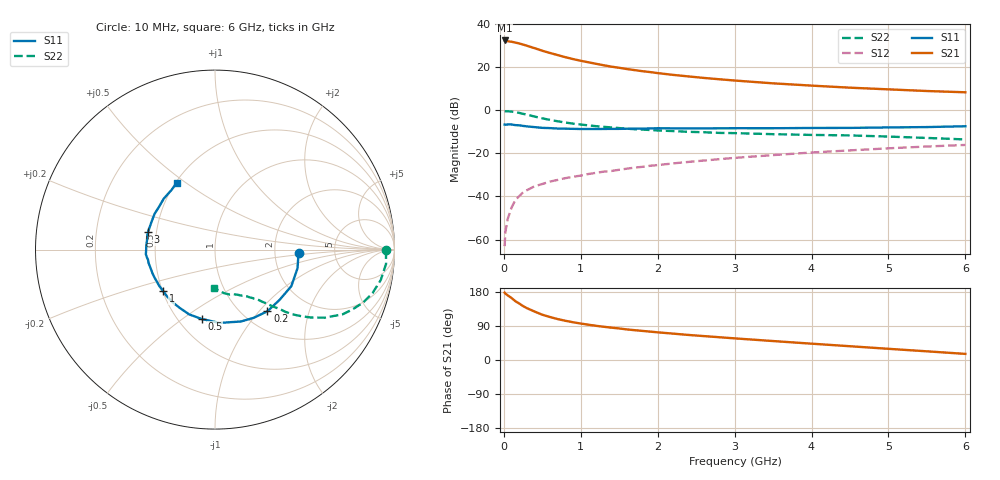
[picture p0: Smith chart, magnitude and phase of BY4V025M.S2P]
! SIEMENS Small Signal Semiconductors
! BFY420
! Si NPN RF SIEGET Grounded Emitter Transistor in MICRO-X
! VCE = 4 V  IC = 25 mA
! Common Emitter S-Parameters:  October  1996
# GHz  S  MA  R  50
!  f  S11  S21  S12  S22
! GHz  MAG  ANG  MAG  ANG  MAG  ANG  MAG  ANG
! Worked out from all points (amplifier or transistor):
!   36 points, 10 MHz to 6 GHz, reference 50 ohm
!   highest |S21| = 32.5 dB at 10 MHz (marker M1)
!   |S21| within 3 dB of that: start of sweep to 348.3 MHz
!   unconditionally stable (mu >= 1): start of sweep to 14.18 MHz; 1.92 GHz to end of sweep
!   at 250 MHz: K = 0.35, MSG = 34.3 dB, |S12| = -38.1 dB
!   at 1.4 GHz: K = 0.94, MSG = 24.2 dB, |S12| = -28.1 dB
!   at 6 GHz: K = 1.06, MAG = 10.8 dB, |S12| = -16.0 dB
!   S11 on the Smith chart (normalised r, x): 10 MHz: 2.76, -0.13; 200 MHz: 1.29, -1.11; 500 MHz: 0.65, -0.59; 1 GHz: 0.50, -0.27; 3 GHz: 0.45, +0.10; 6 GHz: 0.51, +0.46
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0.01  0.4692 -2.3  42.32 177.8  0.0007 67.7  0.9503 -0.2
0.02  0.4657 -5.1  41.78 175.2  0.0015 77.6  0.9528 -1.3
0.05  0.4714 -12.7  40.52 170.7  0.003 84.9  0.9564 -4.8
0.1  0.4716 -25.6  39.54 163.6  0.0055 79.1  0.939 -10.4
0.15  0.4558 -38.0  37.77 155.2  0.0083 74.1  0.9107 -15.4
0.2  0.4511 -49.6  36.07 149.1  0.0102 73.2  0.8772 -19.6
0.25  0.437 -60.4  33.97 142.3  0.0125 68.0  0.8348 -23.6
0.3  0.4257 -70.2  31.93 136.8  0.014 66.4  0.797 -26.9
0.4  0.4093 -86.4  27.99 127.8  0.0173 63.6  0.7197 -31.8
0.5  0.3936 -100.9  24.4 119.5  0.0195 61.5  0.6551 -35.3
0.6  0.3885 -111.8  21.66 113.4  0.0222 61.3  0.6023 -37.9
0.7  0.3795 -121.5  19.34 108.0  0.0243 61.3  0.5598 -40.0
0.8  0.3766 -129.5  17.27 103.5  0.0267 59.5  0.523 -41.5
1  0.37 -141.6  14.26 96.2  0.0306 60.3  0.4702 -43.5
1.1  0.3707 -147.1  13.15 93.1  0.0333 61.2  0.4491 -44.7
1.6  0.3752 -166.3  9.16 80.7  0.0443 60.9  0.3764 -48.8
2.2  0.3834 179.9  6.705 69.6  0.0587 59.8  0.3317 -53.7
3  0.386 165.4  4.957 57.1  0.079 55.9  0.2969 -59.8
3.5  0.3858 157.0  4.263 50.0  0.0916 52.7  0.2806 -63.6
4.5  0.3928 142.3  3.379 36.3  0.1179 44.6  0.2626 -72.2
5.5  0.4105 126.5  2.827 22.9  0.145 35.8  0.2294 -84.3
6  0.4292 119.5  2.641 16.1  0.1578 31.1  0.2118 -92.1
